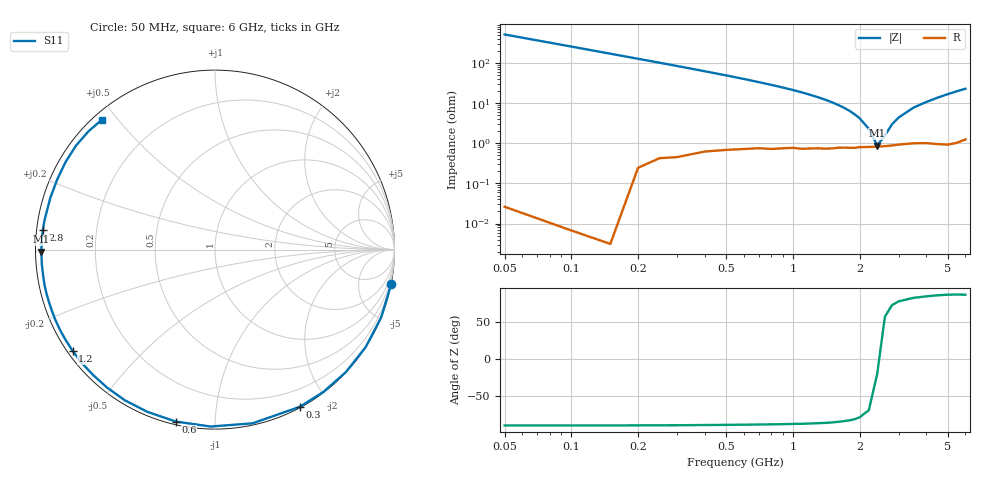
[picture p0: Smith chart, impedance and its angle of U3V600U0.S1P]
! SIEMENS Discrete & RF Semiconductors
! BBY53-02W
! Si Tuning Diode in SCD-80
! VR = 0.6 V
! S-Parameters:  September  1997
# GHz  S  MA  R  50
!  f  S11
! GHz  MAG  ANG
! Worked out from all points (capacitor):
!   34 points, 50 MHz to 6 GHz, reference 50 ohm
!   read as one part to ground: C = 6.24 pF near 50 MHz
!   lowest |Z| = 879 mohm at 2.4 GHz (marker M1)
!   series resonance near 2.438 GHz, so ESL is about 680 pH
!   S11 on the Smith chart (normalised r, x): 50 MHz: 0, -10; 300 MHz: 0.01, -1.67; 600 MHz: 0.01, -0.80; 1.2 GHz: 0.01, -0.32; 2.8 GHz: 0.02, +0.06; 6 GHz: 0.02, +0.45
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0.05  1 -11.2
0.1  1 -22.2
0.15  1 -32.9
0.2  0.9987 -43.1
0.25  0.9967 -52.7
0.3  0.9953 -61.7
0.4  0.9902 -77.8
0.5  0.9861 -91.4
0.6  0.9826 -102.9
0.7  0.9794 -112.7
0.8  0.9784 -120.9
0.9  0.9761 -128.1
1  0.9743 -134.2
1.1  0.9747 -139.7
1.2  0.9734 -144.6
1.4  0.9726 -152.8
1.6  0.9705 -159.7
1.9  0.97 -168.2
2.2  0.9683 -175.1
2.4  0.9676 -179.3
2.8  0.9655 173.5
3  0.9639 170.2
3.5  0.9618 162.6
4  0.9622 156.0
4.5  0.9652 149.5
5  0.9673 143.1
5.5  0.965 136.9
6  0.9596 131.2
